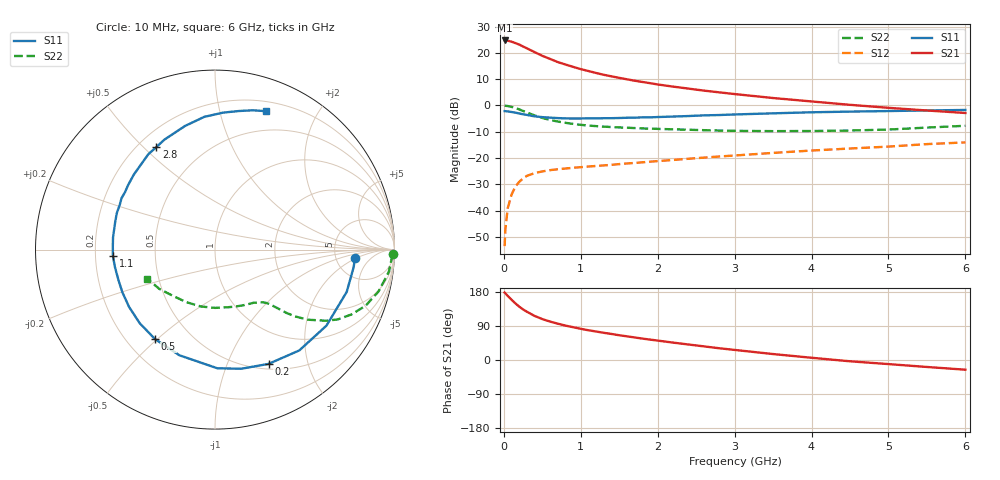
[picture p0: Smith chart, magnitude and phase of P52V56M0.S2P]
! SIEMENS Small Signal Semiconductors
! BFP183
! Si NPN RF Bipolar Junction Transistor in SOT143
! VCE = 2.5 V  IC = 6 mA
! Common Emitter S-Parameters:  March  1996
# GHz  S  MA  R  50
!  f  S11  S21  S12  S22
! GHz  MAG  ANG  MAG  ANG  MAG  ANG  MAG  ANG
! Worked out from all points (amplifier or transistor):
!   36 points, 10 MHz to 6 GHz, reference 50 ohm
!   highest |S21| = 24.7 dB at 10 MHz (marker M1)
!   |S21| within 3 dB of that: start of sweep to 299.5 MHz
!   unconditionally stable (mu >= 1): 1.424 GHz to 5.572 GHz
!   at 250 MHz: K = 0.23, MSG = 25.1 dB, |S12| = -27.8 dB
!   at 1.4 GHz: K = 0.99, MSG = 16.8 dB, |S12| = -22.6 dB
!   at 6 GHz: K = 0.95, MSG = 5.6 dB, |S12| = -14.1 dB
!   lowest NFmin = 1.20 dB at 450 MHz
!   S11 on the Smith chart (normalised r, x): 10 MHz: 7.67, -1.88; 200 MHz: 0.56, -1.42; 500 MHz: 0.32, -0.49; 1.1 GHz: 0.27, -0.03; 2.8 GHz: 0.27, +0.55; 6 GHz: 0.29, +1.39
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0.01  0.7812 -3.5  17.28 177.9  0.0021 78.2  0.9908 -1.5
0.02  0.7787 -7.2  17.17 176.1  0.0044 85.2  0.9857 -2.9
0.05  0.7708 -17.8  17.13 169.1  0.011 84.0  0.9764 -7.3
0.1  0.7517 -34.3  16.36 159.0  0.0201 73.0  0.9408 -14.3
0.15  0.7323 -50.1  15.41 149.4  0.0286 65.8  0.8959 -20.4
0.2  0.7031 -64.9  14.44 140.8  0.0352 59.9  0.8422 -25.4
0.25  0.6798 -77.6  13.26 133.4  0.0409 54.7  0.786 -29.7
0.3  0.6612 -88.9  12.22 127.4  0.0458 50.0  0.7334 -32.7
0.4  0.6213 -108.6  10.36 116.3  0.0516 43.8  0.6476 -37.1
0.5  0.6003 -123.8  8.818 108.0  0.0556 39.3  0.5794 -39.9
0.6  0.5866 -135.6  7.7 101.4  0.0587 37.1  0.5299 -41.6
0.7  0.5756 -146.2  6.71 95.9  0.0611 35.2  0.4949 -42.6
0.9  0.5642 -162.2  5.432 86.6  0.0652 33.7  0.4461 -44.3
1.1  0.5698 -176.5  4.521 78.4  0.0689 33.4  0.4146 -45.9
1.5  0.5777 164.0  3.354 65.3  0.0766 33.7  0.382 -50.0
1.8  0.5944 151.2  2.804 56.5  0.0828 34.5  0.3656 -54.1
2.2  0.6158 137.3  2.285 45.9  0.0918 34.6  0.3518 -60.8
2.8  0.6579 119.8  1.778 31.0  0.1069 33.9  0.3335 -73.0
3.5  0.7088 103.6  1.386 15.7  0.1252 31.9  0.3248 -89.9
4.5  0.7645 86.6  1.029 -3.4  0.1517 26.8  0.3337 -118.8
5.5  0.8039 74.9  0.803 -18.4  0.184 21.3  0.3797 -144.8
6  0.8214 69.9  0.719 -25.6  0.1983 17.2  0.4107 -156.8
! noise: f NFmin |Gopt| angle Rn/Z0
0.45  1.2  0.21  41  0.24
0.9  1.25  0.24  101  0.21
1.8  2  0.32  175  0.14
